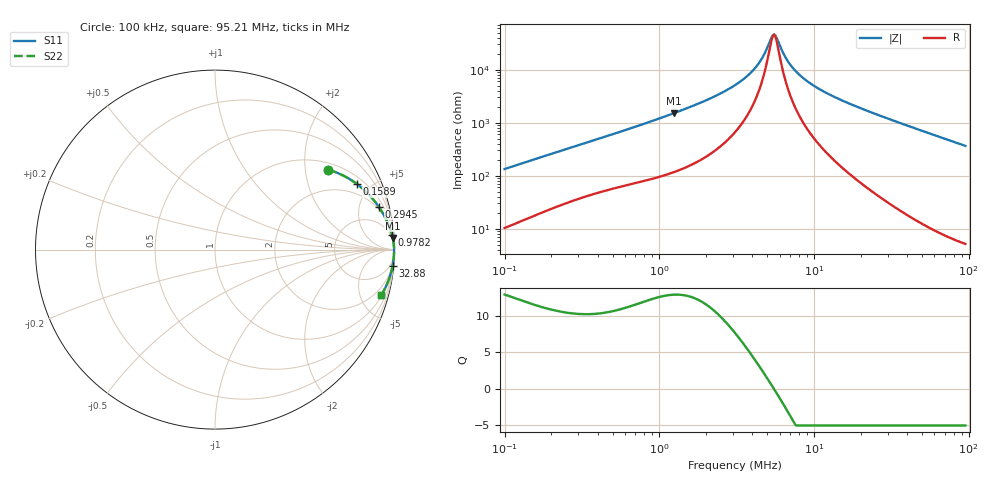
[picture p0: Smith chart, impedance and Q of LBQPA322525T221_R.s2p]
! LBQPA322525T221_R  S-PARAMETER MODEL  ( General Type )
! Model Generated by TAIYO YUDEN Corporation (http://www.ty-top.com)
! Version 1.0
! TAIYO YUDEN Control No. 191025NI43SB-FBB
! Copyright(c) 2019 TAIYO YUDEN CO.,LTD. All Rights Reserved.
! Product Description (link to TY-COMPAS)
! https://ds.yuden.co.jp/TYCOMPAS/or/detail?pn=LBQPA322525T221KR&u=M
! Products Name : Inductors
! Characteristics :
!  Inductance : 220 uH , SRF(min) : 3.0 MHz , DC Resistance(max) : 3.25 Ohm
!  Rated Current : Saturation :190 mA , Temp Rise : 170 mA (20 degC)
!  Case Size : 3.2 x 2.5 / 0.126 x 0.098 [mm/inch] , Thickness : 2.5 / 0.098 [mm/inch]
!  (Conditions: Temperature = 25 degC , DC Bias Current/Voltage = 0A / 0V)
! External Node Assignments :
!  1  o---GGG---o  2
! GND o---------o GND
! Frequency Range : 0.1MHz  -  95.211795MHz  [ 402 STEP ]
# MHz S RI R 50
! Freq[MHz].  S11 Real  S11 Imag  S21 Real  S21 Imag  S12 Real  S12 Imag  S22 Real  S22 Imag
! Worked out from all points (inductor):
!   401 points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, 100 kHz to 95.21 MHz, reference 50 ohm
!   read as one part in series: L = 209 uH near 103.5 kHz
!   highest Q = 12.9 at 1.244 MHz (marker M1), where L = 193 uH
!   self-resonance near 5.434 MHz
!   S11 on the Smith chart (normalised r, x): 100 kHz: 1.21, +2.66; 158.9 kHz: 1.36, +4.14; 294.5 kHz: 1.72, +7.36; 978.2 kHz: 3, +23; 32.88 MHz: 2, -22; 95.21 MHz: 1.10, -7.31
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0.1  0.6312 0.4453  0.3688 -0.4453  0.3688 -0.4453  0.6312 0.4453
0.158877  0.7919 0.3646  0.2081 -0.3646  0.2081 -0.3646  0.7919 0.3646
0.29454  0.9118 0.2391  0.0882 -0.2391  0.0882 -0.2391  0.9118 0.2391
0.31545  0.9201 0.2267  0.0799 -0.2267  0.0799 -0.2267  0.9201 0.2267
0.978171  0.9862 0.0832  0.0138 -0.0832  0.0138 -0.0832  0.9862 0.0832
0.995088  0.9866 0.0818  0.0134 -0.0818  0.0134 -0.0818  0.9866 0.0818
1.243566  0.9906 0.065  0.00936 -0.065  0.00936 -0.065  0.9906 0.065
2.116008  0.9957 0.0349  0.00435 -0.0349  0.00435 -0.0349  0.9957 0.0349
3.085641  0.9971 0.0193  0.00291 -0.0193  0.00291 -0.0193  0.9971 0.0193
3.726142  0.9975 0.0127  0.00252 -0.0127  0.00252 -0.0127  0.9975 0.0127
4.273987  0.9977 0.00812  0.00234 -0.00812  0.00234 -0.00812  0.9977 0.00812
4.737111  0.9978 0.00481  0.00225 -0.00481  0.00225 -0.00481  0.9978 0.00481
5.341222  0.9978 0.000993  0.00217 -0.000993  0.00217 -0.000993  0.9978 0.000993
5.527568  0.9978 -9.15e-05  0.00216 9.15e-05  0.00216 9.15e-05  0.9978 -9.15e-05
5.720415  0.9978 -0.00118  0.00215 0.00118  0.00215 0.00118  0.9978 -0.00118
6.449925  0.9979 -0.00499  0.00214 0.00499  0.00214 0.00499  0.9979 -0.00499
7.14883  0.9978 -0.00832  0.00217 0.00832  0.00217 0.00832  0.9978 -0.00832
9.733658  0.9976 -0.019  0.00242 0.019  0.00242 0.019  0.9976 -0.019
15.20166  0.9965 -0.0379  0.00349 0.0379  0.00349 0.0379  0.9965 -0.0379
30.70484  0.9906 -0.0847  0.00943 0.0847  0.00943 0.0847  0.9906 -0.0847
32.88468  0.9894 -0.091  0.0106 0.091  0.0106 0.091  0.9894 -0.091
95.21179  0.9273 -0.2527  0.0727 0.2527  0.0727 0.2527  0.9273 -0.2527
